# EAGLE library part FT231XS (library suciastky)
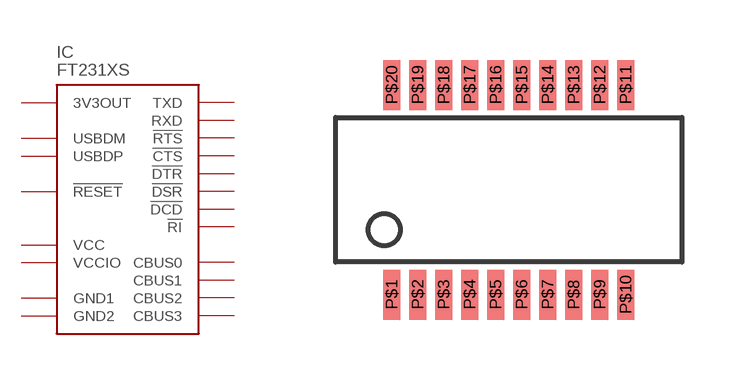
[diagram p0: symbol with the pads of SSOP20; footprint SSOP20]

Designator prefix IC

## FT231XS  [SSOP20]
P$1  !DTR
P$2  !RTS
P$3  VCCIO  pwr
P$4  RXD  in
P$5  !RI
P$6  GND1  pwr
P$7  !DSR
P$8  !DCD
P$9  !CTS
P$10  CBUS2
P$11  USBDP
P$12  USBDM
P$13  3V3OUT  pwr
P$14  !RESET  in
P$15  VCC  pwr
P$16  GND2  pwr
P$17  CBUS1
P$18  CBUS0
P$19  CBUS3
P$20  TXD  out

## Footprint SSOP20 (pad centres in mm)
smd 0.42 x 1.25: P$1 -2.925,-2.625; P$2 -2.275,-2.625; P$3 -1.625,-2.625; P$4 -0.975,-2.625; P$5 -0.325,-2.625; P$6 0.325,-2.625; P$7 0.975,-2.625; P$8 1.625,-2.625; P$9 2.275,-2.625; P$10 2.925,-2.625; P$11 2.925,2.625; P$12 2.275,2.625; P$13 1.625,2.625; P$14 0.975,2.625; P$15 0.325,2.625; P$16 -0.325,2.625; P$17 -0.975,2.625; P$18 -1.625,2.625; P$19 -2.275,2.625; P$20 -2.925,2.625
